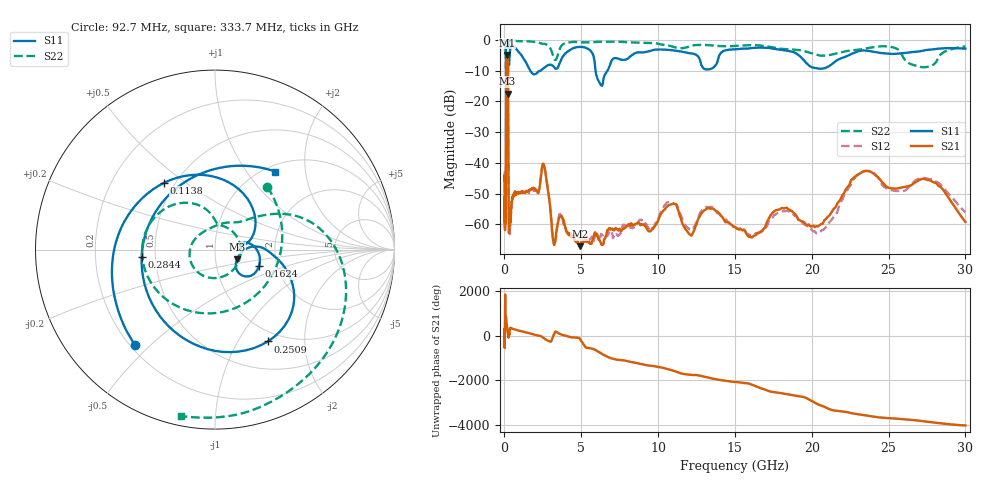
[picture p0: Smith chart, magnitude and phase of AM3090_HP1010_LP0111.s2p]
! Date/Time: Thu, Feb 28, 2019 2:04 PM
! Network Analyzer: Agilent Technologies E8364B Rev: A.07.50.67
! Sweep from 0.010 to 30.000 GHz, 1601 Points, Sweep Type: LOG
! Power Supply: 5.023 V, 0.002 A
# Hz S DB R 50
!freq MagS11 AngS11 MagS21 AngS21 MagS12 AngS12 MagS22 AngS22
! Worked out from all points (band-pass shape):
!   1601 points, 10 MHz to 30 GHz, reference 50 ohm
!   highest |S21| = -4.95 dB at 166.5 MHz (marker M1); lowest = -67.1 dB at 4.903 GHz (marker M2)
!   |S21| within 3 dB of the highest: 127.8 MHz to 220.3 MHz (92.48 MHz wide, 53.1 % of centre)
!   lowest |S11| = -17.4 dB at 199.3 MHz (marker M3), VSWR 1.31, Z = 63.5 - j7.09 ohm
!   |S11| at or under -10 dB: 123 MHz to 223.6 MHz (100.6 MHz wide, 58 % of centre); 1.677 GHz to 2.354 GHz (677 MHz wide, 33.6 % of centre); 5.927 GHz to 6.71 GHz (783.4 MHz wide, 12.4 % of centre)
!   |S22| runs from -18.6 to -0.2 dB; largest |S21 - S12| = 0.012
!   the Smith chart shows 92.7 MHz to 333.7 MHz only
!   S11 on the Smith chart (normalised r, x): 92.7 MHz: 0.22, -0.45; 113.8 MHz: 0.44, +0.41; 162.4 MHz: 1.61, -0.32; 250.9 MHz: 0.86, -1.35; 284.4 MHz: 0.42, -0.04; 333.7 MHz: 1.11, +1.38
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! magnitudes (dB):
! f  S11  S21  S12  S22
! 10 MHz  -0.3  -46.0  -42.7  -0.6
! 38.04 MHz  -0.5  -61.8  -59.1  -1.4
! 48.37 MHz  -0.7  -48.4  -50.0  -1.5
! 92.7 MHz  -3.2  -51.0  -51.0  -6.8
! 113.8 MHz  -6.6  -20.0  -19.9  -7.9
! 144.7 MHz  -14.1  -5.4  -5.4  -17.1
! 162.4 MHz  -11.6  -5.0  -4.9  -16.5
! 166.5 MHz  -11.7  -4.9  -4.9  -16.2
! 199.3 MHz  -17.4  -5.6  -5.6  -18.5
! 228.2 MHz  -9.0  -10.6  -10.5  -12.2
! 250.9 MHz  -4.6  -33.4  -33.5  -2.9
! 284.4 MHz  -7.7  -59.3  -61.1  -1.0
! 333.7 MHz  -5.2  -60.2  -61.6  -0.5
! 550.5 MHz  -2.0  -50.9  -51.0  -0.3
! 2.084 GHz  -10.9  -49.1  -49.2  -0.7
! 2.558 GHz  -9.1  -40.6  -40.5  -1.3
! 3.204 GHz  -8.7  -66.3  -65.5  -5.8
! 4.903 GHz  -2.3  -67.1  -65.1  -0.8
! 7.926 GHz  -6.3  -60.9  -60.2  -0.7
! 20.41 GHz  -9.3  -60.7  -63.0  -5.0
! 23.48 GHz  -3.5  -42.6  -42.7  -2.8
! 30 GHz  -2.8  -59.2  -56.1  -2.2
